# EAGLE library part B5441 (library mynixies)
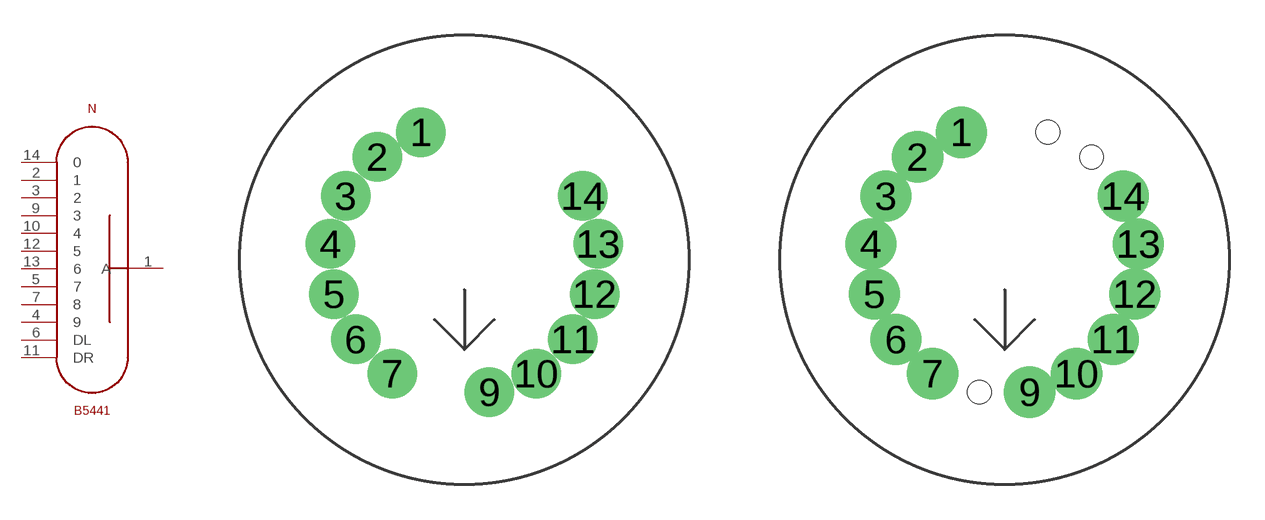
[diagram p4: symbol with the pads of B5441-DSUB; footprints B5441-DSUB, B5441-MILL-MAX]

Designator prefix N

## B5441  [B5441-DSUB]
1  A  pas
2  1  pas
3  2  pas
4  9  pas
5  7  pas
6  DL  pas
7  8  pas
9  3  pas
10  4  pas
11  DR  pas
12  5  pas
13  6  pas
14  0  pas

## B54410339  [B5441-MILL-MAX]
Pads as for B5441-DSUB

## B54410339-1  [B5441-MILL-MAX1]
Pads as for B5441-DSUB

## Footprint B5441-DSUB (pad centres in mm)
drill 1.4 pad 1.8: 1 -1.837,5.412; 2 -3.693,4.362; 3 -5.034,2.705; 4 -5.675,0.672; 5 -5.527,-1.455; 6 -4.609,-3.379; 7 -3.05,-4.833; 9 1.066,-5.615; 10 3.05,-4.833; 11 4.609,-3.379; 12 5.527,-1.455; 13 5.675,0.672; 14 5.034,2.705

## Footprint B5441-MILL-MAX (pad centres in mm)
drill 1.45 pad 1.8: 1 -1.837,5.412; 2 -3.693,4.362; 3 -5.034,2.705; 4 -5.675,0.672; 5 -5.527,-1.455; 6 -4.609,-3.379; 7 -3.05,-4.833; 9 1.066,-5.615; 10 3.05,-4.833; 11 4.609,-3.379; 12 5.527,-1.455; 13 5.675,0.672; 14 5.034,2.705
hole 1 at 1.837,5.412
hole 1 at 3.693,4.362
hole 1 at -1.066,-5.615

## Footprint B5441-MILL-MAX1 (pad centres in mm)
drill 1.45 pad 1.8 offset: 1 -1.837,5.412; 2 -3.693,4.362; 3 -5.034,2.705; 4 -5.675,0.672; 5 -5.527,-1.455; 6 -4.609,-3.379; 7 -3.05,-4.833; 9 1.066,-5.615; 10 3.05,-4.833; 11 4.609,-3.379; 12 5.527,-1.455; 13 5.675,0.672; 14 5.034,2.705
hole 1 at 1.837,5.412
hole 1 at 3.693,4.362
hole 1 at -1.066,-5.615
